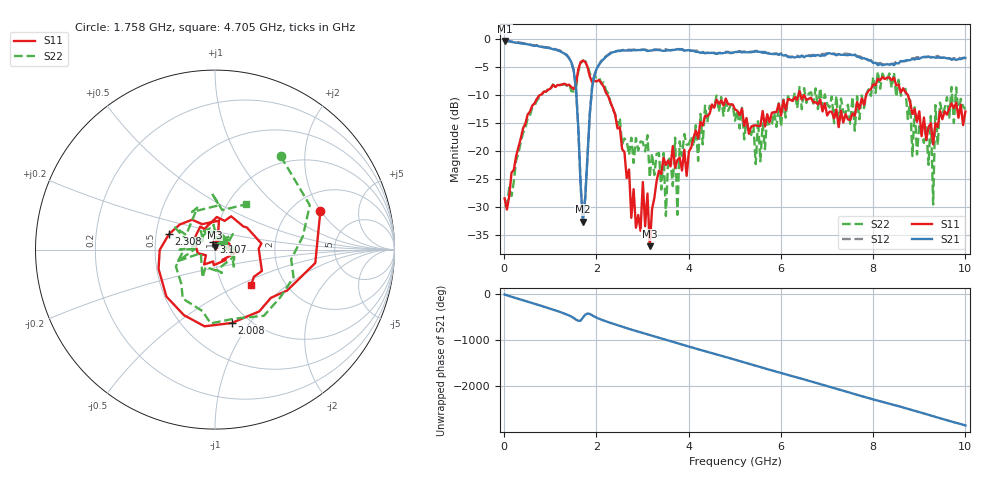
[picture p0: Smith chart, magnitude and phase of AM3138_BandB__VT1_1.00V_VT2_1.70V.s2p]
! Date/Time: Tue, Nov 13, 2018 4:39 PM
! Network Analyzer: Agilent Technologies E8364B Rev: A.07.50.67
! Sweep from 0.010 to 10.000 GHz, 201 Points, Sweep Type: LIN
! Power Supply: 1.000 V, 0.000 A
# Hz S DB R 50
!freq MagS11 AngS11 MagS21 AngS21 MagS12 AngS12 MagS22 AngS22
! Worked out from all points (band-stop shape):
!   201 points, 10 MHz to 10 GHz, reference 50 ohm
!   highest |S21| = -0.31 dB at 10 MHz (marker M1); lowest = -32.6 dB at 1.708 GHz (marker M2)
!   |S21| within 3 dB of the highest: start of sweep to 1.397 GHz; 2.187 GHz to 7.719 GHz (5.533 GHz wide, 112 % of centre)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
!   lowest |S11| = -37.1 dB at 3.157 GHz (marker M3), VSWR 1.03, Z = 49.9 + j1.4 ohm
!   |S11| at or under -10 dB: 2.24 GHz to 6.381 GHz (4.14 GHz wide, 96 % of centre); 6.504 GHz to 7.849 GHz (1.345 GHz wide, 18.7 % of centre); 8.753 GHz to end of sweep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
!   |S22| runs from -31.6 to -3.8 dB; largest |S21 - S12| = 0.031
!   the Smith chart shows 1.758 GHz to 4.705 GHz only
!   S11 on the Smith chart (normalised r, x): 1.758 GHz: 2.79, +2.00; 2.008 GHz: 0.83, -0.83; 2.308 GHz: 0.58, +0.11; 3.107 GHz: 0.98, +0.08; 4.705 GHz: 1.36, -0.59
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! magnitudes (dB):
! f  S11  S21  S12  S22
! 10 MHz  -28.5  -0.3  -0.2  -29.9
! 1.459 GHz  -8.6  -4.2  -4.1  -9.3
! 1.708 GHz  -3.8  -32.6  -32.6  -3.8
! 1.758 GHz  -4.1  -28.4  -28.2  -3.9
! 2.008 GHz  -7.5  -5.2  -5.2  -6.9
! 2.308 GHz  -11.4  -2.5  -2.4  -11.4
! 2.757 GHz  -32.0  -2.0  -1.9  -17.6
! 3.107 GHz  -27.6  -2.1  -2.0  -17.2
! 3.157 GHz  -37.1  -2.1  -1.9  -24.8
! 3.357 GHz  -23.5  -2.0  -1.9  -20.4
! 3.507 GHz  -22.5  -2.1  -1.8  -31.6
! 3.706 GHz  -23.0  -1.9  -1.9  -17.6
! 3.756 GHz  -21.6  -1.8  -1.8  -31.4
! 3.806 GHz  -21.2  -1.9  -1.8  -18.3
! 4.705 GHz  -11.0  -2.5  -2.4  -10.3
! 5.005 GHz  -12.6  -2.3  -2.2  -14.6
! 6.703 GHz  -11.3  -2.9  -2.8  -11.5
! 8.352 GHz  -6.8  -4.5  -4.6  -6.1
! 9.251 GHz  -15.0  -3.3  -3.2  -13.7
! 9.301 GHz  -18.8  -3.2  -3.0  -29.6
! 9.351 GHz  -15.0  -3.3  -3.1  -11.8
! 10 GHz  -12.9  -3.4  -3.3  -12.5
